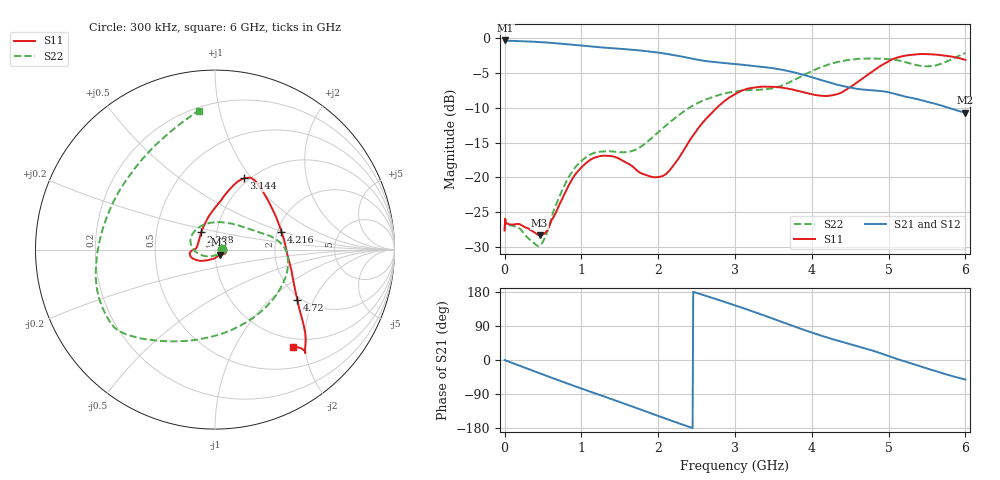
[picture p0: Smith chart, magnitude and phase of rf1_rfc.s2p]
!Agilent Technologies,M9375A,MY55441453,A.02.50.04
!Agilent M9375A: A.02.50.04
!Date: Monday, December 12, 2016 11:32:37
!Correction: S11(Full 2 Port(1,2))
!S21(Full 2 Port(1,2))
!S12(Full 2 Port(1,2))
!S22(Full 2 Port(1,2))
!S2P File: Measurements: S11, S21, S12, S22:
# Hz S  dB  R 50
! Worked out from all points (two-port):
!   751 points, 300 kHz to 6 GHz, reference 50 ohm
!   highest |S21| = -0.38 dB at 8.3 MHz (marker M1); lowest = -10.7 dB at 6 GHz (marker M2)
!   |S21| within 3 dB of the highest: start of sweep to 2.653 GHz
!   lowest |S11| = -28.3 dB at 456.3 MHz (marker M3), VSWR 1.08, Z = 52.5 - j3.03 ohm
!   |S11| at or under -10 dB: start of sweep to 2.765 GHz
!   |S22| runs from -29.9 to -2.2 dB; largest |S21 - S12| = 0.004
!   S11 on the Smith chart (normalised r, x): 300 kHz: 1.09, -0.00; 2.208 GHz: 0.84, +0.17; 3.144 GHz: 0.95, +0.92; 4.216 GHz: 2.10, +0.49; 4.72 GHz: 1.90, -1.52; 6 GHz: 0.84, -1.77
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300000  -27.60 -2.4  -0.39 -0.1  -0.39 -0.1  -27.67 0.9
8299600  -25.93 3.3  -0.38 -0.6  -0.37 -0.4  -25.95 2.8
4.562772e8  -28.29 -48.4  -0.60 -35.0  -0.60 -35.0  -29.80 -82.1
5.522724e8  -27.64 -75.6  -0.68 -42.3  -0.67 -42.4  -27.90 -115.3
7.842608e8  -22.30 -128.5  -0.89 -59.6  -0.88 -59.6  -21.02 -162.9
1.00025e9  -18.57 -150.4  -1.12 -75.3  -1.12 -75.3  -17.63 172.2
1.224239e9  -17.00 -164.3  -1.34 -91.3  -1.34 -91.3  -16.34 147.8
1.488226e9  -17.30 -175.1  -1.56 -110.0  -1.56 -110.1  -16.39 111.7
2.0002e9  -19.95 159.8  -2.12 -147.6  -2.12 -147.7  -13.54 35.5
2.20819e9  -18.15 128.4  -2.48 -162.8  -2.48 -162.9  -11.59 21.8
2.59217e9  -11.98 86.6  -3.29 171.1  -3.29 171.1  -8.95 7.6
3.00015e9  -8.07 71.9  -3.75 144.3  -3.75 144.2  -7.70 -9.2
3.144143e9  -7.36 67.9  -3.92 134.3  -3.92 134.2  -7.51 -20.0
3.352132e9  -7.00 63.5  -4.16 119.5  -4.16 119.4  -7.41 -42.4
3.576121e9  -7.08 58.9  -4.50 103.0  -4.50 102.9  -6.99 -72.4
4.0001e9  -8.09 37.4  -5.64 72.4  -5.64 72.3  -4.77 -117.8
4.216089e9  -8.32 15.1  -6.36 58.3  -6.36 58.3  -3.83 -129.7
4.720064e9  -5.37 -31.6  -7.46 29.3  -7.46 29.2  -2.97 -144.3
5.00005e9  -3.34 -42.5  -7.80 10.2  -7.79 10.1  -3.05 -154.7
5.416029e9  -2.33 -48.9  -8.90 -16.9  -8.90 -17.0  -4.01 164.2
5.720014e9  -2.54 -48.5  -9.81 -36.0  -9.81 -36.2  -3.56 122.0
6e9  -3.16 -51.3  -10.73 -51.6  -10.73 -51.7  -2.17 96.8
